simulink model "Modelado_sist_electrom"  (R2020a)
settings: Solver=VariableStepAuto  StartTime=0.0  StopTime=10.0  RelTol=1e-3
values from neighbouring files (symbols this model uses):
  b = 0.1    [Comando_linmod.m]
  k = 0.8    [Comando_linmod.m]
  kf = 0.45    [Comando_linmod.m]
  kv = 0.45    [Comando_linmod.m]
  L = 0.1    [Comando_linmod.m]
  m = 0.15    [Comando_linmod.m]
  M = 5    [Comando_linmod.m]
  R = 0.25    [Comando_linmod.m]
  v = 5    [Comando_linmod.m]

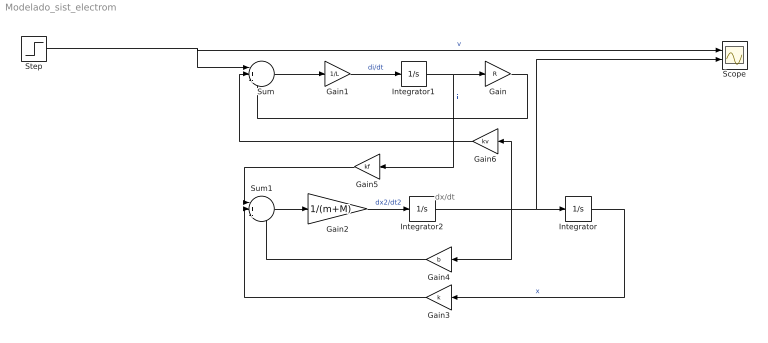
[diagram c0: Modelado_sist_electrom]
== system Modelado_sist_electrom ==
  note: dx/dt
  Gain : Gain  Gain=R
  Gain1 : Gain  Gain=1/L
  Gain2 : Gain  Gain=1/(m+M)
  Gain3 : Gain  Gain=k
  Gain4 : Gain  Gain=b
  Gain5 : Gain  Gain=kf
  Gain6 : Gain  Gain=kv
  Integrator : Integrator
  Integrator1 : Integrator
  Integrator2 : Integrator
  Scope : Scope  NumInputPorts=2
  Step : Step  After=v  SampleTime=0
  Sum : Sum  Inputs=|+--
  Sum1 : Sum  Inputs=|+--
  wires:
  Gain1/1 -> Integrator1/1  "di/dt"
  Gain3/1 -> Sum1/2
  Sum1/1 -> Gain2/1
  Gain4/1 -> Sum1/3
  Integrator2/1 -> Gain4/1, Gain6/1, Scope/2, Integrator/1
  Gain6/1 -> Sum/2
  Integrator/1 -> Gain3/1  "x"
  Gain2/1 -> Integrator2/1  "dx2/dt2"
  Gain/1 -> Sum/3
  Step/1 -> Sum/1, Scope/1  "v"
  Gain5/1 -> Sum1/1
  Integrator1/1 -> Gain5/1, Gain/1  "i"
  Sum/1 -> Gain1/1
